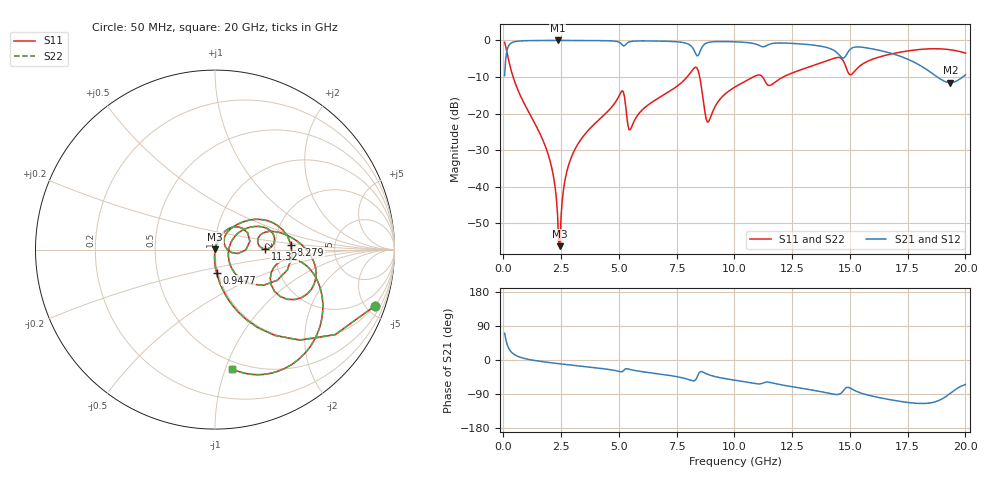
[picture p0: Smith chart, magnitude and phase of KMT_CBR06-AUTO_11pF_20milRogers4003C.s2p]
! Data measured by Modelithics Inc. support@modelithics.com 813-866-6335
! KEMET CBR06-AUTO 11pF, Pad Width= 0.851mm, Pad Length= 0.64mm, Pad Gap= 0.62mm, 20mil Rogers 4003C substrate Data, January 2022
# hz S ma R 50
! 2 Port Network Data from SP1.SP block
! freq  magS11  angS11  magS21  angS21  magS12  angS12  magS22  angS22
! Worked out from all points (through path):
!   401 points, 50 MHz to 20 GHz, reference 50 ohm
!   highest |S21| = -0.01 dB at 2.344 GHz (marker M1); lowest = -11.5 dB at 19.35 GHz (marker M2)
!   group delay of S21, straight-line fit = 16.9 ps
!   lowest |S11| = -56.3 dB at 2.444 GHz (marker M3), VSWR 1.00, Z = 50.1 + j0.107 ohm
!   |S11| at or under -10 dB: 418.8 MHz to 7.952 GHz (7.533 GHz wide, 180 % of centre); 8.495 GHz to 10.81 GHz (2.319 GHz wide, 24 % of centre); 11.22 GHz to 12.11 GHz (897.4 MHz wide, 7.69 % of centre)
!   |S22| runs from -56.3 to -0.5 dB; largest |S21 - S12| = 0
!   S11 on the Smith chart (normalised r, x): 50 MHz: 0.98, -5.68; 947.8 MHz: 0.98, -0.26; 8.279 GHz: 2.47, +0.15; 11.32 GHz: 1.77, +0.01; 20 GHz: 0.44, -1.06
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5e7  0.9443 -19.4  0.3289 70.6  0.3289 70.6  0.9443 -19.4
3.4925e8  0.3737 -69.4  0.9271 20.5  0.9271 20.5  0.3737 -69.4
9.4775e8  0.1281 -86.2  0.9911 3.5  0.9911 3.5  0.1281 -86.2
1.995125e9  0.02387 -94.9  0.9988 -6.8  0.9988 -6.8  0.02387 -94.9
2.34425e9  0.004055 -86.9  0.999 -9.4  0.999 -9.4  0.004055 -86.9
2.444e9  0.001535 44.1  0.999 -10.1  0.999 -10.1  0.001535 44.1
2.793125e9  0.01841 74.5  0.9988 -12.5  0.9988 -12.5  0.01841 74.5
3.391625e9  0.04592 72.0  0.9976 -16.5  0.9976 -16.5  0.04592 72.0
5.087375e9  0.1955 36.7  0.9095 -31.2  0.9095 -31.2  0.1955 36.7
5.486375e9  0.05994 28.3  0.9629 -25.1  0.9629 -25.1  0.05994 28.3
6.73325e9  0.1642 51.0  0.9798 -36.7  0.9798 -36.7  0.1642 51.0
8.279375e9  0.425 3.4  0.7068 -54.5  0.7068 -54.5  0.425 3.4
8.52875e9  0.2775 -44.0  0.7275 -30.7  0.7275 -30.7  0.2775 -44.0
8.877875e9  0.07718 1.9  0.9397 -38.6  0.9397 -38.6  0.07718 1.9
1.0025e10  0.2306 32.6  0.957 -53.5  0.957 -53.5  0.2306 32.6
1.132175e10  0.2781 0.7  0.8298 -59.0  0.8298 -59.0  0.2781 0.7
1.336662e10  0.4482 7.2  0.8662 -79.3  0.8662 -79.3  0.4482 7.2
1.4414e10  0.5809 -14.2  0.691 -91.0  0.691 -91.0  0.5809 -14.2
1.496262e10  0.3467 -27.4  0.7252 -72.8  0.7252 -72.8  0.3467 -27.4
1.670825e10  0.6442 -22.7  0.6764 -104.4  0.6764 -104.4  0.6442 -22.7
1.935162e10  0.745 -69.0  0.2647 -87.6  0.2647 -87.6  0.745 -69.0
2e10  0.6717 -81.7  0.3374 -64.8  0.3374 -64.8  0.6717 -81.7
